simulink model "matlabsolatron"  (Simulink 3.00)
settings: Solver=ode1  SolverMode=SingleTasking  StartTime=0.0  StopTime=inf  RelTol=1e-3
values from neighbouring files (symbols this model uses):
  h = 0.01    [design.m]    (also in initfra.m; initlab1.m; tst.m)
undefined symbols (not defined in the file or in its folder): solatron_settings

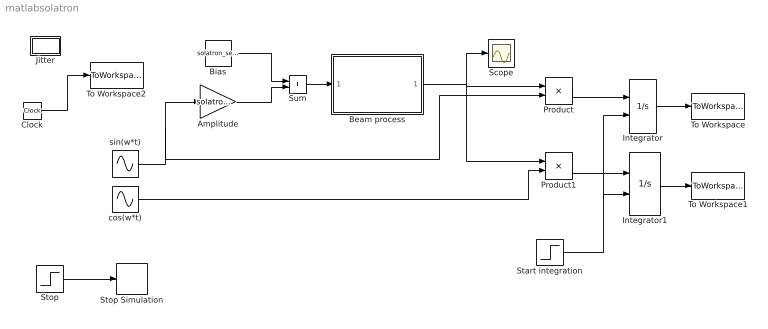
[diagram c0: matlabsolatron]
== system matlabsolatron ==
  Amplitude : Gain  Gain=solatron_settings.u0  SaturateOnIntegerOverflow=on
  Beam process : Subsystem
  Bias : Constant  Value=solatron_settings.bias
  Clock : Clock
  Integrator : Integrator  ExternalReset=rising  InitialConditionSource=internal  InitialCondition=0  LimitOutput=off  UpperSaturationLimit=inf  LowerSaturationLimit=-inf  ShowSaturationPort=off  ShowStatePort=off  AbsoluteTolerance=auto
  Integrator1 : Integrator  ExternalReset=rising  InitialConditionSource=internal  InitialCondition=0  LimitOutput=off  UpperSaturationLimit=inf  LowerSaturationLimit=-inf  ShowSaturationPort=off  ShowStatePort=off  AbsoluteTolerance=auto
  Jitter : Subsystem
  Product : Product  Inputs=2  SaturateOnIntegerOverflow=on
  Product1 : Product  Inputs=2  SaturateOnIntegerOverflow=on
  Scope : Scope
  Start integration : Step  Time=solatron_settings.Tstart  Before=0  After=1  SampleTime=h
  Stop : Step  Time=solatron_settings.Tstop  Before=0  After=1  SampleTime=0
  Stop Simulation : Stop
  Sum : Sum  Inputs=++  SaturateOnIntegerOverflow=on
  To Workspace : ToWorkspace  VariableName=s_T  SampleTime=-1  SaveFormat=Matrix
  To Workspace1 : ToWorkspace  VariableName=c_T  SampleTime=-1  SaveFormat=Matrix
  To Workspace2 : ToWorkspace  VariableName=time  SampleTime=-1  SaveFormat=Matrix
  cos(w*t) : Sin  Amplitude=1  Frequency=solatron_settings.w  Phase=pi/2  SampleTime=0
  sin(w*t) : Sin  Amplitude=1  Frequency=solatron_settings.w  Phase=0  SampleTime=0
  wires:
  Product/1 -> Integrator/1
  Product1/1 -> Integrator1/1
  cos(w*t)/1 -> Product1/2
  Integrator/1 -> To Workspace/1
  Integrator1/1 -> To Workspace1/1
  sin(w*t)/1 -> Product/2, Amplitude/1
  Sum/1 -> Beam process/1(In1)
  Amplitude/1 -> Sum/2
  Bias/1 -> Sum/1
  Start integration/1 -> Integrator1/2, Integrator/2
  Beam process/1(Out1) -> Product/1, Product1/1, Scope/1
  Stop/1 -> Stop Simulation/1
  Clock/1 -> To Workspace2/1

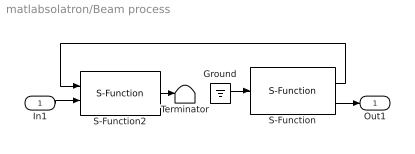
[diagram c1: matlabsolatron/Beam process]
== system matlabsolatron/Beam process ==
  In1 : Inport  Port=1  PortWidth=-1  SampleTime=-1  DataType=auto
  Ground : Ground
  S-Function : S-Function  FunctionName=analogin  Parameters=solatron_settings.h [0]  PortCounts=[]  SFunctionModules=''
  S-Function2 : S-Function  FunctionName=analogout  Parameters=solatron_settings.h [0]  PortCounts=[]  SFunctionModules=''
  Terminator : Terminator
  Out1 : Outport  Port=1
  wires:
  Ground/1 -> S-Function/1
  S-Function2/1 -> Terminator/1
  S-Function/1 -> S-Function2/1
  S-Function/2 -> Out1/1
  In1/1 -> S-Function2/2

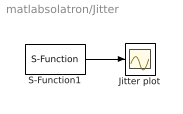
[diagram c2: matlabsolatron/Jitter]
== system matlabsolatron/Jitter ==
  Jitter plot : Scope
  S-Function1 : S-Function  FunctionName=timer  Parameters=solatron_settings.h  PortCounts=[]  SFunctionModules=''
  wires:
  S-Function1/1 -> Jitter plot/1
